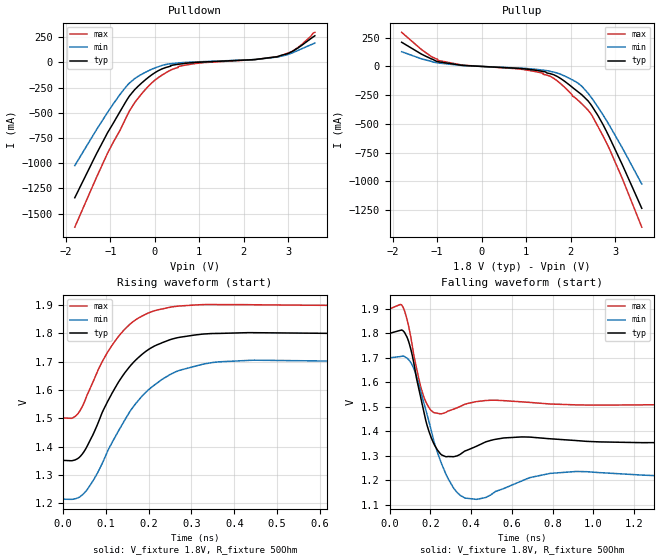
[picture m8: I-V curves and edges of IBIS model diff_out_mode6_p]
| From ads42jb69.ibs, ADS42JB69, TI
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|   diff_out_mode6 Model
[Model]   diff_out_mode6_p
Model_type   Output
Polarity   Non-Inverting
Vmeas = 1.589
Vref = 1.8
Cref = 0.5pF
Rref = 50
|   typ   min   max
|   (nom PVT)   (fast PVT)   (slow PVT)
C_comp   2.834e-12   2.356e-12   2.851e-12
[Model spec]
|subparameter   typ   min   max
Vmeas   1.589   1.49   1.7074
| Where nom  PVT is Nominal Process, 1.8V, 25C
|   Fast PVT is Strong Process,  1.9V, -40C
|   Slow PVT is Weak Process,   1.7V, 125C
[Voltage Range]   1.8   1.7   1.9
|Junction Temperature
[Temperature Range]   25   125   -40
[Pullup Reference]   1.8   1.7   1.9
[Pulldown Reference]   0   0   0
[Power Clamp Reference]   1.8   1.7   1.9
[GND Clamp Reference]   0   0   0
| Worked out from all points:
|   slope of the pulldown table from 0 to 0.27 V, typ, clamps not added: 4.94 ohm
|   slope of the pullup table from 0 to 0.27 V, typ, clamps not added: 49.4 ohm
|   falling waveform, V_fixture 1.8V, R_fixture 50Ohm: 20-80 % time 67.1ps typ, 95.6ps min, 56.3ps max; typ from 1.8 V to 1.35 V
|   rising waveform, V_fixture 1.8V, R_fixture 50Ohm: 20-80 % time 102ps typ, 118ps min, 91.1ps max; typ from 1.35 V to 1.8 V
[Pulldown]
|   Voltage   I(typ)   I(min)   I(max)
-1.8V     -1.341A    -1.023A    -1.633A
-1.063V   -697.3mA   -495.9mA   -900.2mA
-613.8mV  -362.2mA   -224.7mA   -518.5mA
-373.1mV  -235.8mA   -138.1mA   -353.7mA
20.08fV   -102.9mA   -55.72mA   -177.1mA
358.2mV   -31.82mA   -13.52mA   -76.66mA
621mV     -13.42mA   -2.427mA   -32.54mA
1.082V    3.463mA    7.44mA     -3.434mA
2.252V    27.83mA    28.39mA    27.17mA
2.842V    70.11mA    61.5mA     65.03mA
3.213V    140.7mA    117mA      145.1mA
3.6V      263.4mA    191mA      297.7mA
[Pullup]
|   Voltage   I(typ)   I(min)   I(max)
-1.8V     210.2mA    128.1mA    296.7mA
-1.323V   100.9mA    62.84mA    137.7mA
-986.8mV  40.99mA    30.49mA    52.6mA
-450mV    9.747mA    7.957mA    12.52mA
1.082V    -26.39mA   -20.41mA   -36.01mA
1.374V    -43.31mA   -32.15mA   -58.84mA
1.705V    -88.58mA   -58.29mA   -127.7mA
2.154V    -217mA     -142.8mA   -290.2mA
2.483V    -347.4mA   -279.5mA   -428.4mA
2.865V    -610.5mA   -507.9mA   -710.8mA
3.182V    -871.6mA   -722.3mA   -993.5mA
3.6V      -1.234A    -1.023A    -1.399A
[Ramp]
R_load = 50
|   typ   min   max
dV/dt_r   0.112302/5.91733e-11   0.147577/7.37194e-11  0.0911225/4.77257e-11
dV/dt_f   0.267621/6.70643e-11   0.290297/9.55807e-11   0.236283/5.62284e-11
[Falling Waveform]
V_fixture = 1.8V
V_fixture_min = 1.7V
V_fixture_max = 1.9V
R_fixture = 50Ohm
|   Time   V(typ)   V(min)   V(max)
0s        1.799V     1.699V     1.899V
58ps      1.813V     1.706V     1.916V
88ps      1.778V     1.696V     1.847V
152ps     1.539V     1.564V     1.582V
196ps     1.392V     1.43V      1.493V
284ps     1.297V     1.212V     1.481V
372ps     1.32V      1.128V     1.511V
560ps     1.373V     1.167V     1.525V
914ps     1.362V     1.236V     1.508V
2.258ns   1.353V     1.215V     1.505V
[Rising Waveform]
V_fixture = 1.8V
V_fixture_min = 1.7V
V_fixture_max = 1.9V
R_fixture = 50Ohm
|   Time   V(typ)   V(min)   V(max)
0s        1.352V     1.215V     1.502V
32ps      1.356V     1.218V     1.511V
56ps      1.399V     1.247V     1.58V
82ps      1.483V     1.31V      1.669V
106ps     1.564V     1.39V      1.737V
164ps     1.696V     1.54V      1.841V
200ps     1.743V     1.601V     1.872V
250ps     1.778V     1.655V     1.892V
348ps     1.8V       1.697V     1.902V
2.16ns    1.798V     1.698V     1.899V
